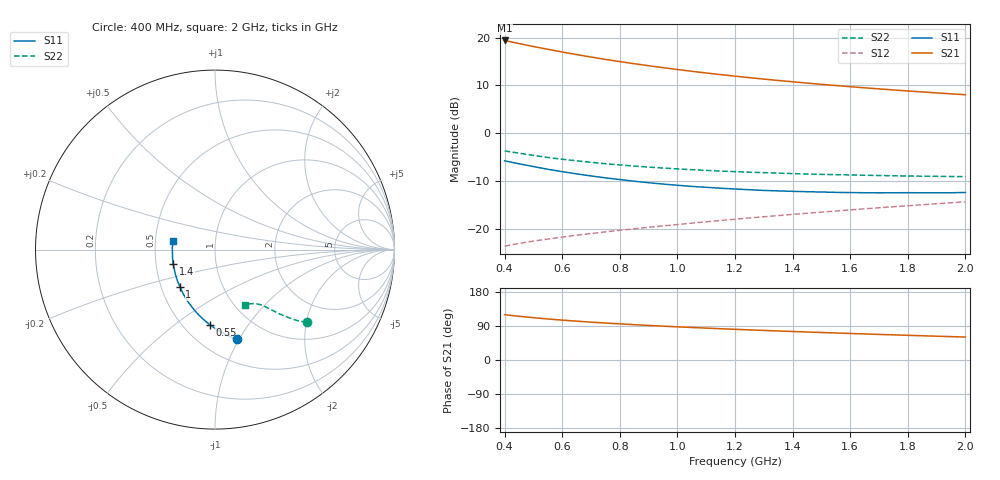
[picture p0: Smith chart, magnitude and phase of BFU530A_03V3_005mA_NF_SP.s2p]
! Filename:  P:\Prog\Test\Noise\ATS_data\Testdata_Net\06 Compressed Noise after Statistics\BFU530A_APG2013_33_A05_03p3V_005mA_NF_CM01_D.sf
! Date/Time: Tue 16/Apr/2013 15:11:04
! BFU530A_APG2013_33_A05_03p3V_1to25mA_NF_CM01_Bias4_R.sf
! Noise Parameter Data File
! BFU530A_APG2013_33_A05_03p3V_1to25mA_NF_CM01
! Date/time: Fri Apr 12 14:21:19 2013
! VAR V_out= 3.301000
! VAR I_out= 5.000000
! VAR V_in= 0.823300
! VAR I_in= 0.053905
! Device data file deembeded for feedlines and parallel
! Original file: \06 Compressed Noise after Statistics\BFU530A_APG2013_33_A05_03p3V_005mA_NF_CM01_R.sf
! Feed-files: PR017V01_150413_Feed1.s2p, PR017V01_150413_Feed2.s2p
! Parallel-file: PR017V01_150413_Par.s2p
# MHz S MA R 50
!  Freq-MHz  S11-mag  S11-arg  S21-mag  S21-arg  S12-mag  S12-arg  S22-mag  S22-arg
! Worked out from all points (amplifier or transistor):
!   37 points, 400 MHz to 2 GHz, reference 50 ohm
!   highest |S21| = 19.4 dB at 400 MHz (marker M1)
!   |S21| within 3 dB of that: start of sweep to 654 MHz
!   unconditionally stable (mu >= 1): 1.591 GHz to end of sweep
!   at 500 MHz: K = 0.61, MSG = 20.4 dB, |S12| = -22.6 dB
!   at 1.1 GHz: K = 0.92, MSG = 15.6 dB, |S12| = -18.6 dB
!   at 2 GHz: K = 1.02, MAG = 10.4 dB, |S12| = -14.4 dB
!   lowest NFmin = 0.60 dB at 460 MHz
!   S11 on the Smith chart (normalised r, x): 400 MHz: 0.72, -0.98; 550 MHz: 0.67, -0.68; 1 GHz: 0.62, -0.28; 1.4 GHz: 0.62, -0.11; 2 GHz: 0.62, +0.07
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400  0.5132 -76.2  9.335 119.6  0.06566 59.6  0.6528 -38.3
420  0.499 -78.8  9.062 117.8  0.06751 59.2  0.6378 -39.1
460  0.4715 -83.8  8.539 114.7  0.07096 58.6  0.611 -40.5
500  0.4472 -88.5  8.066 111.7  0.07421 58.1  0.5857 -41.6
550  0.4188 -94.1  7.551 108.2  0.07794 57.7  0.5566 -42.8
600  0.3953 -99.2  7.068 105.2  0.08175 57.6  0.5334 -43.8
650  0.375 -104.0  6.64 102.5  0.08548 57.5  0.5135 -44.7
700  0.3568 -108.7  6.262 99.9  0.08903 57.5  0.4951 -45.4
750  0.3405 -113.1  5.915 97.6  0.09262 57.7  0.4788 -46.0
800  0.3271 -117.5  5.609 95.3  0.09625 57.9  0.4652 -46.6
850  0.3142 -121.7  5.33 93.2  0.09984 58.0  0.4522 -47.2
900  0.303 -125.8  5.076 91.2  0.1035 58.2  0.4414 -47.7
950  0.2932 -129.7  4.846 89.3  0.107 58.5  0.4315 -48.3
1000  0.2849 -133.4  4.635 87.5  0.1107 58.7  0.4227 -48.7
1100  0.2712 -140.8  4.263 84.2  0.1181 59.2  0.4077 -49.7
1200  0.2604 -147.7  3.949 81.0  0.1257 59.5  0.3956 -50.8
1300  0.2516 -154.2  3.68 78.0  0.1334 59.9  0.3861 -51.8
1400  0.2462 -160.6  3.446 75.2  0.1412 60.1  0.3775 -53.0
1500  0.2422 -166.7  3.242 72.6  0.1492 60.3  0.3705 -54.2
1650  0.2379 -174.9  2.983 68.8  0.1615 60.4  0.363 -56.3
1750  0.2377 179.7  2.833 66.3  0.1698 60.5  0.3581 -57.6
2000  0.2394 168.0  2.524 60.6  0.1912 60.2  0.3508 -61.5
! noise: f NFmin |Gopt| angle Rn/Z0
400  0.6403  0.173  28.72  0.1125
460  0.603  0.1606  38.77  0.1046
600  0.7086  0.1688  31.96  0.1235
800  0.6936  0.1478  68.89  0.0948
1000  0.7041  0.1476  83.12  0.0931
1200  0.7677  0.1537  98.05  0.091
1400  0.7821  0.178  121.8  0.0805
1600  0.8226  0.1763  134.3  0.0763
1800  0.8193  0.2175  148.8  0.064
2000  0.8238  0.2302  171.8  0.0603
